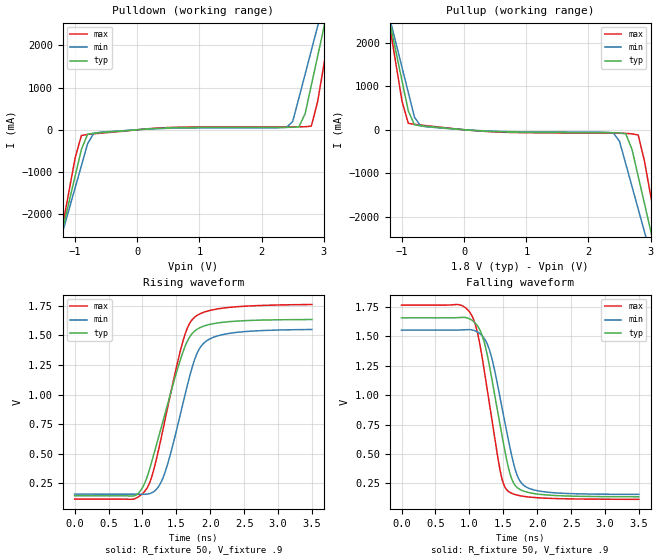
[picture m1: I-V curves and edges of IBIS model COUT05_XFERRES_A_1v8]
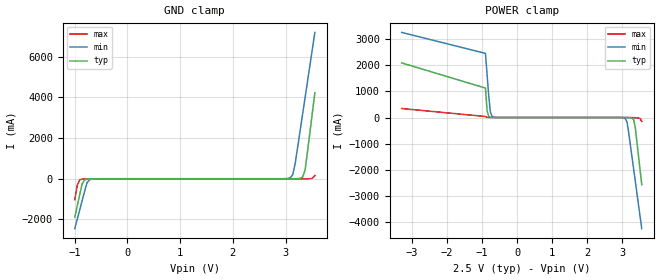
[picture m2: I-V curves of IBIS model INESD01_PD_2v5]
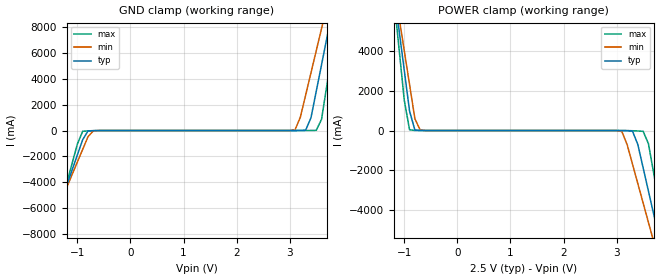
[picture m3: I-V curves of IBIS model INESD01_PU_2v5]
|   This file is an IBIS representation of the   |
|   Integrated Device Technology , Inc.   |
|   ICS83026I   |
|   LOW SKEW, 1-TO-2 DIFFERENTIAL-TO-LVCMOS/LVTTL FANOUT BUFFER   |
[IBIS Ver]   4.1
[File name]   83026i_01.ibs
[File Rev]   1.0
[Date]   24 Nov 2009 | Last modified
|   Aug 22 2003 | Generated
[Source]   Originated at Integrated Device Technology, Inc.
[Disclaimer]
IDT hereby grants the user of this IBIS model a non-exclusive,
nontransferable license to use this IBIS model under the following terms.
Before using this IBIS model, the user should read this license.
If the user does not accept these terms,  the IBIS model should be
returned to IDT within 30 days.
   The user is granted this license only to use the IBIS model and
is not granted rights to sell, load, rent, lease or license the IBIS
model in whole or in part, or in modified form to anyone other than
user. User may modify the IBIS model to suit its specific
applications but rights to derivative works and such modifications
shall belong to IDT.
   This IBIS model is provided on an "AS IS" basis and IDT makes
absolutely no warranty with respect to the information contained
herein. IDT DISCLAIMS AND CUSTOMER WAIVES ALL WARRANTIES, EXPRESS
OR IMPLIED, INCLUDING WARRANTIES OF MERCHANTABILITY OR FITNESS FOR
A PARTICULAR PURPOSE. The entire risk as to quality and performance
is with the Customer. ACCORDINGLY, IN NO EVENT SHALL THE COMPANY BE
LIABLE FOR ANY DAMAGES, WHETHER IN CONTRACT OR TORT,INCLUDING ANY
LOST PROFITS OR OTHER INCIDENTAL, CONSEQUENTIAL, EXEMPLARY, OR
PUNITIVE DAMAGES ARISING OUT OF THE USE OR APPLICATION OF THE IBIS
model provided in this package. Further, IDT reserves the right to
make changes without notice to any product herein to improve
reliability, function, or design. IDT does not convey any license
under patent rights or any other intellectual property rights,
including those of third parties.
   IDT is not obligated to provide maintenance or support
for the licensed IBIS model.
[Copyright]   Copyright 2003 by Integrated Device Technology , Inc.
[Component]   ICS83026MI-01
[Manufacturer] Integrated Device Technology, Inc.
[Package]
|SOIC 8 Lead
|   typ   min   max
R_pkg   57.05m   55.5m   58.6m
L_pkg   1.769nH   1.570nH   1.968nH
C_pkg   0.269pF   0.252pF   0.286pF
[Pin]   signal_name   model_name   R_pin   L_pin   C_pin
1   VDD   POWER   58.6m   1.968n   0.286p
2   CLK   INESD01_PD   55.5m   1.570n   0.252p
3   nCLK   INESD01_PU   55.5m   1.570n   0.252p
4   OE   INESD01_PU   56.6m   1.968n   0.286p
5   GND   GND   58.6m   1.968n   0.286p
6   Q1   COUT05_XFERRES_A   55.5m   1.570n   0.252p
7   Q0   COUT05_XFERRES_A   55.5m   1.570n   0.252p
8   VDDO   POWER   56.6m   1.968n   0.286p
[Diff Pin]   inv_pin  vdiff tdelay_typ tdelay_min  tdelay_max
2   3   NA   0   0   0
[Component]   ICS83026GI-01
[Manufacturer] Integrated Device Technology, Inc.
[Package]
|TSSOP 8 Lead
|   typ   min   max
R_pkg   52.5m   48.8m   56.2m
L_pkg   1.381nH   1.275nH   1.486nH
C_pkg   0.236pF   0.230pF   0.242pF
[Pin]   signal_name   model_name   R_pin   L_pin   C_pin
1   VDD   POWER   56.2m   1.486n   0.242p
2   CLK   INESD01_PD   48.8m   1.275n   0.230p
3   nCLK   INESD01_PU   48.8m   1.275n   0.230p
4   OE   INESD01_PU   56.2m   1.468n   0.242p
5   GND   GND   56.2m   1.486n   0.242p
6   Q1   COUT05_XFERRES_A   48.8m   1.275n   0.230p
7   Q0   COUT05_XFERRES_A   48.8m   1.275n   0.230p
8   VDDO   POWER   56.2m   1.468n   0.242p
[Diff Pin]   inv_pin  vdiff tdelay_typ tdelay_min  tdelay_max
2   3   NA   0   0   0
[Model Selector] INESD01_PD
INESD01_PD_2v5  Buffer selection for 2v5
INESD01_PD_3v3  Buffer selection for 3v3
[Model Selector] INESD01_PU
INESD01_PU_2v5  Buffer selection for 2v5
INESD01_PU_3v3  Buffer selection for 3v3
[Model Selector] COUT05_XFERRES_A
COUT05_XFERRES_A_1v8  Buffer selection for 1v8
COUT05_XFERRES_A_2v5  Buffer selection for 2v5
COUT05_XFERRES_A_3v3  Buffer selection for 3v3
| Models and submodels in the file (7): COUT05_XFERRES_A_1v8 (Output), INESD01_PD_2v5 (Input), INESD01_PU_2v5 (Input), COUT05_XFERRES_A_2v5 (Output), INESD01_PD_3v3 (Input), INESD01_PU_3v3 (Input), COUT05_XFERRES_A_3v3 (Output)
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[Model] COUT05_XFERRES_A_1v8
Model_type   Output
Polarity   Non-Inverting
|   typ   min   max
C_comp   2pF   1.5pF   2.5pF
Vmeas = .9
Rref = 50
Cref = 0
Vref = .9
|   typ   min   max
[Voltage range]   1.8V   1.710V   1.890V
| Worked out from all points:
|   slope of the pulldown table from 0 to 0.27 V, typ, clamps not added: 9.93 ohm
|   slope of the pullup table from 0 to 0.27 V, typ, clamps not added: 10.3 ohm
|   rising waveform, R_fixture 50, V_fixture .9: 20-80 % time 441ps typ, 371ps min, 385ps max; typ from 0.143 V to 1.64 V
|   falling waveform, R_fixture 50, V_fixture .9: 20-80 % time 294ps typ, 296ps min, 273ps max; typ from 1.66 V to 0.137 V
[Pulldown]
|Voltage   I (typ)   I (min)   I (max)
-3.3V     -15.43A    -13.35A    -18.94A
-1.3V     -2.966A    -2.936A    -3.05A
-1.2V     -2.341A    -2.415A    -2.254A
-900mV    -466.8mA   -850.9mA   -137.6mA
-700mV    -81.98mA   -81.55mA   -96.11mA
2.4V      57.31mA    55.13mA    69.01mA
2.7V      379.5mA    1.316A     70.79mA
2.9V      1.732A     2.445A     656.8mA
3V        2.409A     3.01A      1.521A
3.1V      3.087A     3.576A     2.386A
3.2V      3.766A     4.142A     3.251A
6.6V      27.19A     23.68A     33.13A
[Pullup]
|Voltage   I (typ)   I (min)   I (max)
-3.3V     16.84A     14.54A     20.68A
-1.2V     2.486A     2.567A     2.394A
-900mV    433.7mA    855.2mA    147.7mA
-700mV    91.31mA    86.54mA    108.4mA
2.4V      -68.76mA   -72.93mA   -78.48mA
2.6V      -92.56mA   -784.7mA   -84.91mA
2.8V      -1.069A    -1.82A     -121.6mA
2.9V      -1.69A     -2.339A    -712.8mA
3V        -2.312A    -2.858A    -1.506A
3.1V      -2.934A    -3.377A    -2.3A
3.2V      -3.557A    -3.896A    -3.094A
6.6V      -24.74A    -21.59A    -30.09A
[Ramp]
|   typ   min   max
dV/dt_r   1.195/0.633n   1.116/0.564n   1.319/0.568n
dV/dt_f   1.22/0.436n   1.12/0.445n   1.324/0.399n
R_load =   50.0000
[Rising Waveform]
R_fixture = 50
V_fixture = .9   |Vcc_typ
V_fixture_min = .855 |Vcc_min
V_fixture_max = .945 |Vcc_max
C_fixture = 0.0p
| Time   typ   min   max
0s        142.8mV    156.8mV    114.7mV
879.4ps   142.6mV    156.6mV    116.3mV
1.058ns   286.2mV    156.3mV    199.8mV
1.16ns    478.6mV    174.9mV    349.8mV
1.321ns   815.7mV    322.7mV    754.1mV
1.598ns   1.362V     928.7mV    1.455V
1.773ns   1.539V     1.303V     1.656V
1.906ns   1.58V      1.436V     1.697V
2.144ns   1.609V     1.502V     1.728V
3.497ns   1.635V     1.55V      1.762V
[Falling Waveform]
R_fixture = 50
V_fixture = .9   |Vcc_typ
V_fixture_min = .855 |Vcc_min
V_fixture_max = .945 |Vcc_max
C_fixture = 0.0p
| Time   typ   min   max
0s        1.657V     1.553V     1.765V
840.8ps   1.66V      1.553V     1.769V
1.03ns    1.64V      1.555V     1.683V
1.139ns   1.572V     1.53V      1.48V
1.293ns   1.259V     1.39V      935.9mV
1.464ns   708.6mV    943.8mV    329.1mV
1.573ns   390.2mV    624.2mV    183.8mV
1.71ns    212.9mV    312.1mV    150.2mV
1.874ns   172.7mV    209.4mV    135mV
3.497ns   137mV      157.3mV    115.1mV
[Model] INESD01_PD_2v5
Model_type   Input
Polarity   Non-Inverting
Vinl = 0.8V
Vinh = 2.0V
|   typ   min   max
C_comp   2pF   1.5pF   2.5pF
|   typ   min   max
[Voltage range]  2.5V   2.375V   2.625V
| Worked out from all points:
|   GND clamp passes 1 mA (typ) near -0.55 V on its own axis
|   POWER clamp passes 1 mA (typ) near -0.68 V on its own axis
[GND_clamp]
|Voltage I(typ)   I(min)   I(max)
-1V       -1.886A    -2.451A    -1.028A
-953.5mV  -1.338A    -1.994A    -328mA
-907mV    -789.6mA   -1.537A    -53.04mA
-860.5mV  -251.4mA   -1.081A    -21.51mA
-767.5mV  -17.28mA   -198.8mA   -10.01mA
-674.5mV  -5.28mA    -15.38mA   -3.684mA
3.092V    224.5uA    49.06mA    51.52uA
3.139V    500.8uA    208.3mA    52.98uA
3.185V    1.252mA    774.6mA    56.66uA
3.325V    81.55mA    3.177A     200uA
3.371V    416.9mA    3.978A     464.6uA
3.557V    4.225A     7.185A     159.2mA
[POWER_clamp]
|Voltage   I(typ)   I(min)   I(max)
-3.3V     2.083A     3.246A     343.1mA
-907mV    1.122A     2.445A     37.78mA
-860.5mV  267.5mA    1.644A     5.973mA
-814mV    47.03mA    844mA      1.727mA
-767.5mV  9.66mA     215.3mA    677uA
-674.5mV  960.6uA    12.66mA    131.4uA
3.092V    -1.849mA   -49.09mA   -51.51uA
3.139V    -3.491mA   -186mA     -159.7uA
3.325V    -84.03mA   -1.955A    -5.102mA
3.371V    -365.4mA   -2.411A    -8.31mA
3.51V     -2.01A     -3.782A    -35.44mA
3.557V    -2.558A    -4.239A    -152.3mA
[Model] INESD01_PU_2v5
Model_type   Input
Polarity   Non-Inverting
Vinl = 1.4V
Vinh = 1.85V
|   typ   min   max
C_comp   2pF   1.5pF   2.5pF
|   typ   min   max
[Voltage range]  2.5V   2.375V   2.625V
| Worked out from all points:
|   GND clamp passes 1 mA (typ) near -0.54 V on its own axis
|   POWER clamp passes 1 mA (typ) near -0.66 V on its own axis
[GND_clamp]
|Voltage   I(typ)   I(min)   I(max)
-2.5V     -19.6A     -17.18A    -23.67A
-1.6V     -8.969A    -8.332A    -10.1A
-1.5V     -7.788A    -7.349A    -8.588A
-900mV    -707.1mA   -1.46A     -57.43mA
-700mV    -7.027mA   -24.05mA   -13.28mA
3.1V      199.2uA    53.94mA    11.78uA
3.3V      28.4mA     2.748A     652.4uA
3.5V      3.045A     6.192A     15.72mA
3.6V      5.115A     7.914A     872.4mA
3.7V      7.185A     9.638A     3.52A
3.9V      11.33A     13.09A     8.818A
5V        34.14A     32.07A     37.99A
[POWER_clamp]
|Voltage   I(typ)   I(min)   I(max)
-1.5V     9.257A     9.207A     9.48A
-1.2V     7.185A     7.484A     6.83A
-1.1V     5.115A     5.761A     4.182A
-900mV    976.9mA    2.318A     34.23mA
-700mV    1.582mA    24.31mA    1.044mA
3.1V      -2.107mA   -51.03mA   -534.5uA
3.3V      -35.62mA   -1.705A    -10.86mA
3.5V      -1.886A    -3.666A    -39.41mA
3.6V      -3.066A    -4.647A    -666.9mA
3.8V      -5.426A    -6.612A    -3.684A
3.9V      -6.607A    -7.595A    -5.193A
5V        -19.6A     -18.41A    -21.79A
